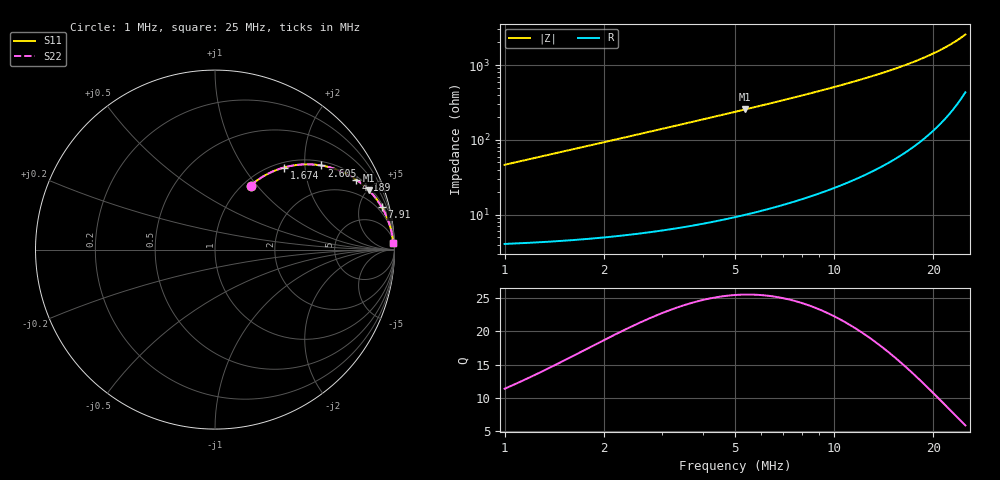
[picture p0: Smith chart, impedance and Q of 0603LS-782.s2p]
# MHz S MA R 50
!Freq  MagS11  AngS11  MagS21  AngS21  MagS12  AngS12  MagS22  AngS22
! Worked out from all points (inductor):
!   801 points, 1 MHz to 25 MHz, reference 50 ohm
!   read as one part in series: L = 7.38 uH near 1.016 MHz
!   highest Q = 25.5 at 5.376 MHz (marker M1), where L = 7.56 uH
!   S11 on the Smith chart (normalised r, x): 1 MHz: 1.08, +0.93; 1.674 MHz: 1.09, +1.55; 2.605 MHz: 1.11, +2.43; 4.189 MHz: 1.16, +3.94; 7.91 MHz: 1.32, +7.75; 25 MHz: 10, +50
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1  0.4083 61.0  0.8777 -24.0  0.8777 -24.0  0.4083 61.0
1.165204  0.4616 58.1  0.852 -27.4  0.852 -27.4  0.4616 58.1
1.314695  0.5058 55.6  0.8276 -30.3  0.8276 -30.3  0.5058 55.6
1.673672  0.5971 50.0  0.7673 -36.6  0.7673 -36.6  0.5971 50.0
2.096651  0.6809 44.2  0.6978 -42.8  0.6978 -42.8  0.6809 44.2
2.605476  0.755 38.4  0.6215 -49.0  0.6215 -49.0  0.755 38.4
2.963499  0.7941 35.0  0.5738 -52.5  0.5738 -52.5  0.7941 35.0
3.343702  0.8269 31.9  0.5285 -55.7  0.5285 -55.7  0.8269 31.9
3.742445  0.854 29.1  0.4864 -58.6  0.4864 -58.6  0.854 29.1
4.188739  0.8777 26.4  0.4453 -61.3  0.4453 -61.3  0.8777 26.4
5  0.9086 22.5  0.3836 -65.2  0.3836 -65.2  0.9086 22.5
5.375559  0.9191 21.1  0.3597 -66.7  0.3597 -66.7  0.9191 21.1
6.520788  0.9421 17.5  0.3002 -70.3  0.3002 -70.3  0.9421 17.5
7.909999  0.9588 14.3  0.2473 -73.3  0.2473 -73.3  0.9588 14.3
9.033197  0.9675 12.4  0.2146 -75.2  0.2146 -75.2  0.9675 12.4
10.86984  0.9767 10.0  0.1738 -77.3  0.1738 -77.3  0.9767 10.0
13.02738  0.983 8.0  0.1385 -79.0  0.1385 -79.0  0.983 8.0
17.05826  0.989 5.3  0.0931 -80.6  0.0931 -80.6  0.989 5.3
21.02813  0.9916 3.5  0.06224 -80.5  0.06224 -80.5  0.9916 3.5
22.97439  0.9923 2.8  0.05005 -79.7  0.05005 -79.7  0.9923 2.8
24.70004  0.9927 2.3  0.0404 -78.4  0.0404 -78.4  0.9927 2.3
25  0.9927 2.2  0.03882 -78.1  0.03882 -78.1  0.9927 2.2
